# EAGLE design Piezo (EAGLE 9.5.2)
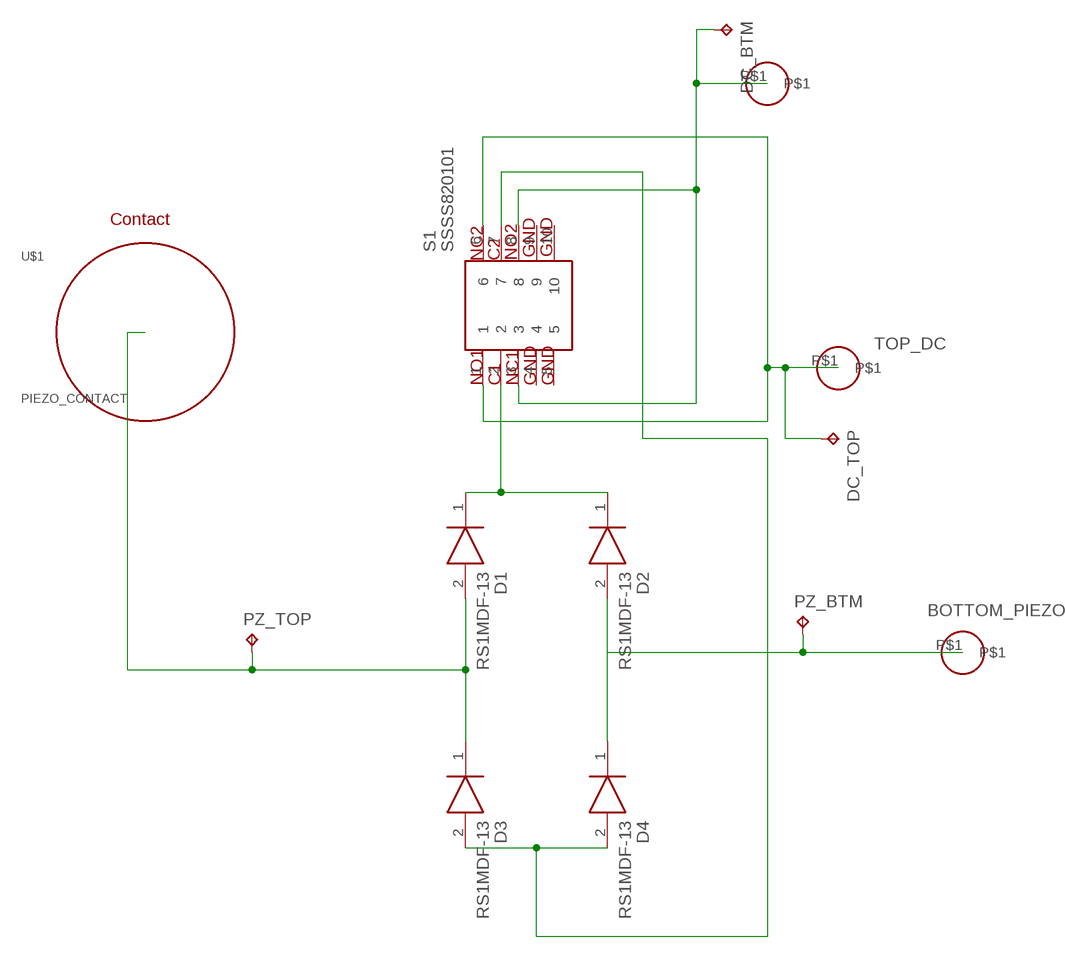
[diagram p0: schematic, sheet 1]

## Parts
D1  RS1MDF-13  [DIOC5327X110N]
D2  RS1MDF-13  [DIOC5327X110N]
D3  RS1MDF-13  [DIOC5327X110N]
D4  RS1MDF-13  [DIOC5327X110N]
DC_BTM  TPB1,27  [B1,27]
DC_TOP  TPB1,27  [B1,27]
PZ_BTM  TPB1,27  [B1,27]
PZ_TOP  TPB1,27  [B1,27]
S1  SSSS820101  [SSSS820101]
U$1  PIEZO_CONTACT  [PIEZO_CONTACT]
U$3  SPRING_PADSINGLE_SIDE  [SPRINGPAD_SINGLE_SIDE]
U$4  SPRING_PADSINGLE_SIDE  [SPRINGPAD_SINGLE_SIDE]
U$5  SPRING_PAD  [SPRING_PAD]

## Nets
BOTTOM_DC [connect]: DC_BTM.TP S1.3 S1.8 U$3.P$1
BOTTOM_PIEZO [connect]: D2.2(A) D4.1(K) PZ_BTM.TP U$4.P$1
N$1 [connect]: D1.1(K) D2.1(K) S1.2
N$2 [connect]: D1.2(A) D3.1(K) PZ_TOP.TP U$1.P$1
N$4 [connect]: D3.2(A) D4.2(A) S1.7
TOP_DC [connect]: DC_TOP.TP S1.1 S1.6 U$5.P$1
Unconnected: S1.4 S1.5 S1.9 S1.10

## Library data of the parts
D1-D4 = RS1MDF-13:RS1MDF-13: Rectifiers Fast Recovery Rectifier; DESCRIPTION: Rectifiers Fast Recovery Rectifier; HEIGHT: 1.1mm; MANUFACTURER_NAME: Diodes Inc.; MANUFACTURER_PART_NUMBER: RS1MDF-13
DC_BTM DC_TOP PZ_BTM PZ_TOP = testpad:TP: Test pad
S1 = RGB_library:SSSS820101: Slide Switches 0.3 Amp at 5 Volts SMD/SMT Source: Datasheet; DESCRIPTION: Slide Switches 0.3 Amp at 5 Volts SMD/SMT; HEIGHT: mm; MANUFACTURER_NAME: ALPS; MANUFACTURER_PART_NUMBER: SSSS820101; MOUSER_PART_NUMBER: 688-SSSS820101; MOUSER_PRICE-STOCK: https://www.mouser.com/Search/Refine.aspx?Keyword=688-SSSS820101
U$1 = RGB_library:PIEZO_CONTACT
U$3-U$5 = RGB_library:SPRING_PAD

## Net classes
1 connect: width 0.457 mm, clearance 0.152 mm

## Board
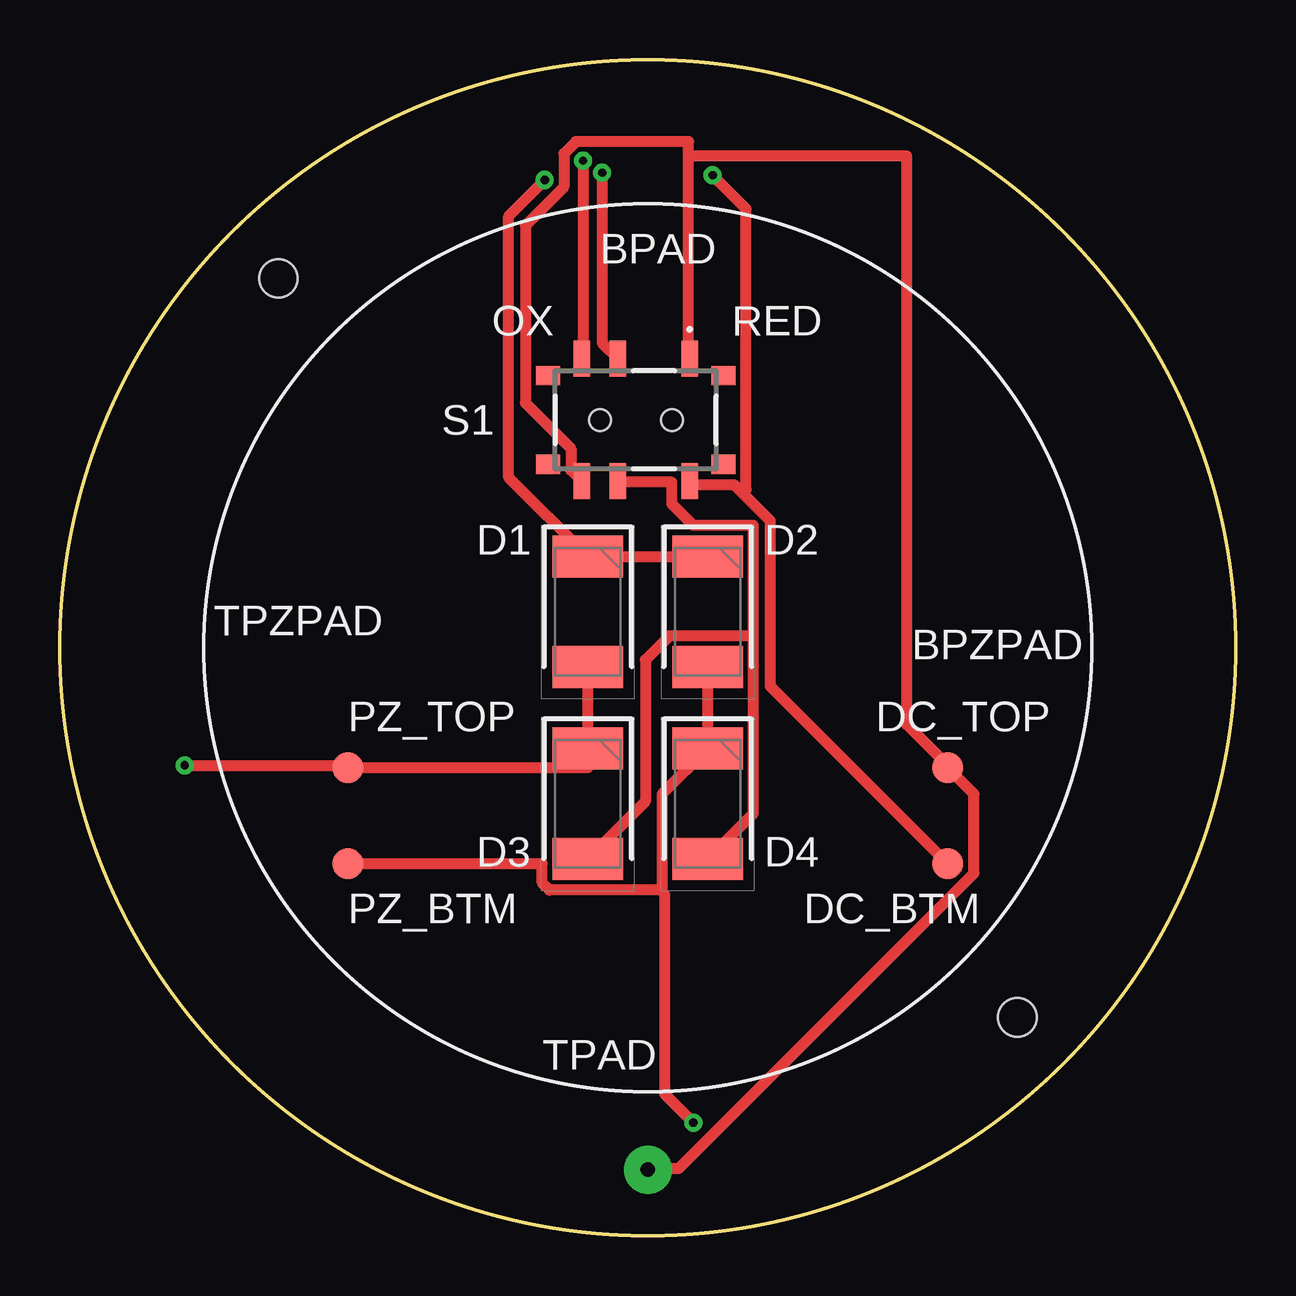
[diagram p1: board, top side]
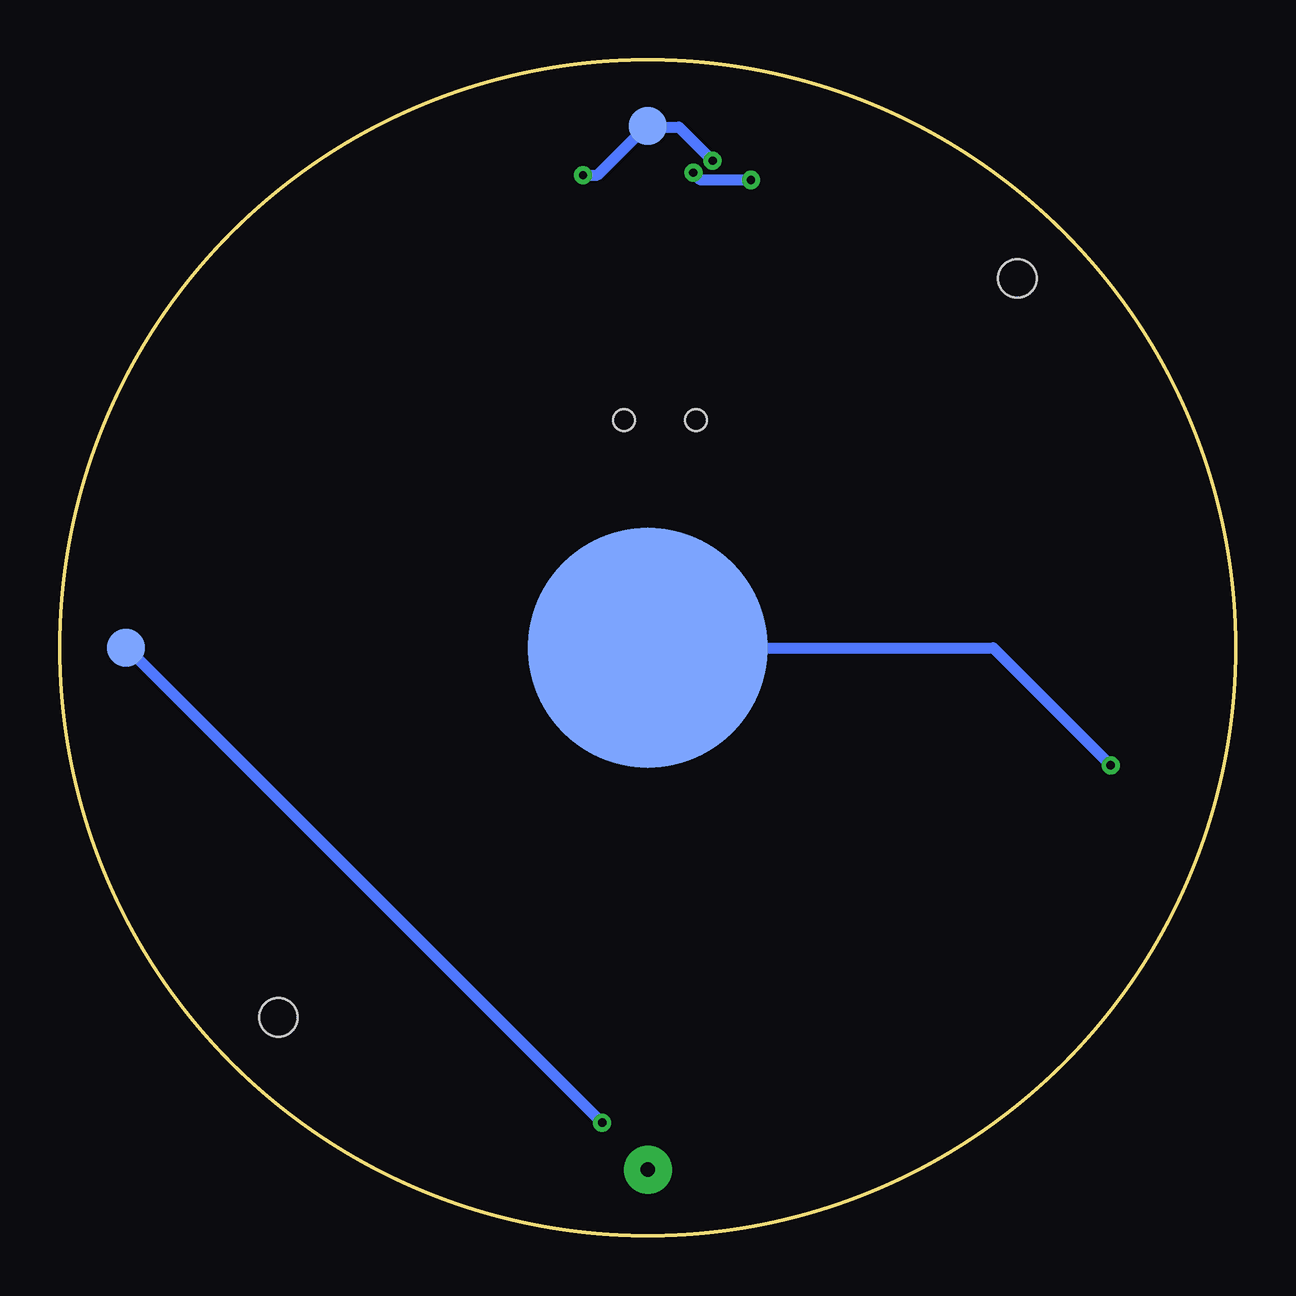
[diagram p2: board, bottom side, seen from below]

Size 49 x 49 mm. Coordinates in mm from the lower left corner, seen from the top.
Outline: circle at 24.5,24.5 radius 24.5
Copper layers (1*16): Top 0.035mm / dielectric 1.5mm / Bottom 0.035mm
Design rules "default *": minimum track width 6mil, minimum drill 0.35mm, track to track 6mil, track to pad 6mil, pad to pad 6mil, via to via 6mil, smd to smd 6mil, copper to edge 40mil, drill to drill 6mil, minimum pad ring 10mil, minimum via ring 8mil, stop-mask expansion 4mil, vias tented up to drill 0mil, thermal gap 10mil
Holes 1.6 mm at 9.1,39.9 39.9,9.1
vRestrict: area 14.5,14.5 to 34.5,34.5

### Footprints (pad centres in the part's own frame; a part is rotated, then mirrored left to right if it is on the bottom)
DIOC5327X110N = smd 1.75 x 2.95: 1 -2.3,0; 2 2.3,0
B1,27 = smd 1.27 x 1.27: TP 0,0
SSSS820101 = smd 0.7 x 1.5: 1 -2.25,-2.55; 2 0.75,-2.55; 3 2.25,-2.55; 6 2.25,2.55; 7 0.75,2.55; 8 -2.25,2.55 | smd 1 x 0.8: 4 3.65,-1.85; 5 3.65,1.85; 9 -3.65,1.85; 10 -3.65,-1.85 | hole 0.9: -1.5,0; 1.5,0
PIEZO_CONTACT = smd 10 x 10: P$1 0,0
SPRINGPAD_SINGLE_SIDE = smd 1.562 x 1.562: P$1 0,0
SPRING_PAD = drill 0.6 pad 2: P$1 0,0

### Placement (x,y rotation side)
D1  22,26 270 top
D2  27,26 270 top
D3  22,18 270 top
D4  27,18 270 top
DC_BTM  37,15.5 0 top
DC_TOP  37,19.5 0 top
PZ_BTM  12,15.5 0 top
PZ_TOP  12,19.5 0 top
S1  24,34 180 top
U$1  24.5,24.5 0 bottom
U$3  24.5,46.25 0 bottom
U$4  46.25,24.5 0 bottom
U$5  24.5,2.75 0 top

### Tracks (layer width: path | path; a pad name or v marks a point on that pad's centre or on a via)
BOTTOM_DC  (via drill 0.35)
  Top 0.457: v21.8,44.8 21.8,36.6 S1.3 | DC_BTM.TP 29.6,22.9 29.6,29.8 28.45,30.95 | 28.45,30.95 28.1,31.3 26.3,31.3 26.3,31.4 S1.8 | v27.2,44.2 28.6,42.8 28.6,31.1 28.45,30.95
  Bottom 0.457: v21.8,44.8 23.2,46.2 24.5,46.2 U$3.P$1 24.7,46.1 26.6,44.2 v27.2,44.2
BOTTOM_PIEZO  (via drill 0.35)
  Top 0.457: PZ_BTM.TP 20.1,15.5 20.1,14.7 20.4,14.4 25.1,14.4 | 25.1,14.4 25.1,18.4 D4.1 D2.2 | v26.4,4.7 25.2,5.9 25.2,14.2 25.1,14.4
  Bottom 0.457: v26.4,4.7 46.2,24.5 U$4.P$1
N$1  (via drill 0.35)
  Top 0.457: S1.2 22.6,37.2 v22.6,44.3 | v20.2,44 18.7,42.5 18.7,31.6 D1.1 D2.1
  Bottom 0.457: v22.6,44.3 22.3,44 v20.2,44
N$2  (via drill 0.35)
  Top 0.457: D1.2 D3.1 22,19.5 PZ_TOP.TP 11.8,19.6 v5.2,19.6
  Bottom 0.457: v5.2,19.6 10.1,24.5 U$1.P$1
N$4
  Top 0.457: 28.9,25 28.9,17.6 D4.2 | 28.9,25 28.9,29.6 26.4,29.6 25.5,30.5 25.5,31.4 23.3,31.4 S1.7 | D3.2 24.4,18.1 24.4,24 25.4,25 28.9,25
TOP_DC
  Top 0.457: S1.6 21.3,31.9 21.3,32.8 19.4,34.7 19.4,42.1 21,43.7 21,45.1 21.5,45.6 26.2,45.6 26.2,45 | 26.2,45 26.2,36.6 S1.1 | U$5.P$1 24.5,2.8 25.8,2.8 38.1,15.1 38.1,18.4 DC_TOP.TP 36.9,19.7 35.3,21.3 35.3,45 26.2,45

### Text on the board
tNames: BPAD | OX | RED | TPZPAD | BPZPAD | TPAD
